(* Logix 5000 AddOnInstructionDefinition export AMCI_SMD34E2_Axis_Follower_Linear; software revision 20.03 *)

ADD_ON_INSTRUCTION AMCI_SMD34E2_Axis_Follower_Linear   (* revision 5.0, vendor AMCI, ExecuteEnableInFalse *)
// Revision note:
// Version 5.0  unlatches the error bit if the rung goes false.  Also modified the Axis Follower commands to by default use the jog CCW command and have an option of the jog CW command.  (The status bits of the jog CCW update faster and the jog CW has smoother motion.)
// Help:
// 2/2017: V0 is the initial release
// 7/2017: V1 added enable and error bits.
// 5/2019: V2 added unlatching the error bit when the rung goes false and the ability to select between normal (jog CCW) and continuous follower (jog CW)
VAR_OUTPUT
   EN : BOOL; {visible}
END_VAR
VAR_INPUT
   Axis_Status_Bits : INT; {required}
   _0_for_Normal_1_for_Continuous : BOOL;
   _0_follow_motor_1_follow_encoder : BOOL;
   Follower_Position : REAL; {required}
   Follower_Velocity : REAL; {required}
   Acceleration : INT; {required}
   Deceleration : INT; {required}
   Proportional_Coefficient : INT; {required}
   Network_delay : INT; {required}
END_VAR
VAR_OUTPUT
   Axis_Follower_occurring : BOOL; {visible}
END_VAR
VAR_IN_OUT
   AMCI_SMD34E2_output_data : _000A:SMD34E2_788832CB:O:0; {required}
END_VAR
VAR_OUTPUT
   ER : BOOL; {visible}
END_VAR
VAR
   command_data_block : INT[10];
        [0]   // Command Bits MSW
        [1]   // Command Bits LSW
        [2]   // Upper Target Position
        [3]   // Lower Target Position
        [4]   // Upper Programmed Speed
        [5]   // Lower Programmed Speed
   axis_follower_position : DINT;
   axis_follower_velocity : DINT;
END_VAR

ROUTINE EnableInFalse   (* ladder *)
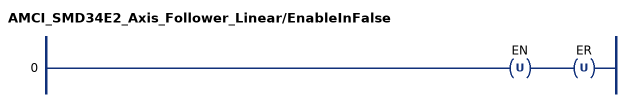
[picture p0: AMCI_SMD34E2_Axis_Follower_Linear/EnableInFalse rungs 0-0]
   0: OTU(EN)OTU(ER);
END_ROUTINE

ROUTINE Logic   (* ladder *)
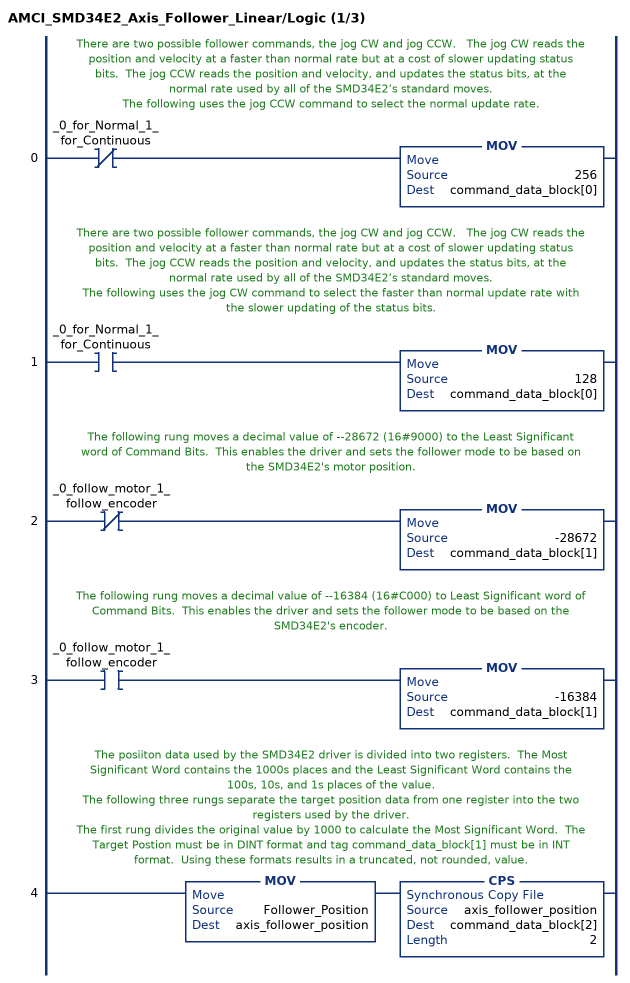
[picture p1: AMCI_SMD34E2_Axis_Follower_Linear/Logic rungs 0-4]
   // There are two possible follower commands, the jog CW and jog CCW.   The jog CW reads the position and velocity at a faster than normal rate but at a cost of slower updating status bits.  The jog CCW reads the position and velocity, and updates the status bits, at the normal rate used by all of the SMD34E2’s standard moves.
   // The following uses the jog CCW command to select the normal update rate.
   0: XIO(_0_for_Normal_1_for_Continuous)MOV(256,command_data_block[0]);
   // There are two possible follower commands, the jog CW and jog CCW.   The jog CW reads the position and velocity at a faster than normal rate but at a cost of slower updating status bits.  The jog CCW reads the position and velocity, and updates the status bits, at the normal rate used by all of the SMD34E2’s standard moves.
   // The following uses the jog CW command to select the faster than normal update rate with the slower updating of the status bits.
   1: XIC(_0_for_Normal_1_for_Continuous)MOV(128,command_data_block[0]);
   // The following rung moves a decimal value of --28672 (16#9000) to the Least Significant word of Command Bits.  This enables the driver and sets the follower mode to be based on the SMD34E2's motor position.
   2: XIO(_0_follow_motor_1_follow_encoder)MOV(-28672,command_data_block[1]);
   // The following rung moves a decimal value of --16384 (16#C000) to Least Significant word of Command Bits.  This enables the driver and sets the follower mode to be based on the SMD34E2's encoder.
   3: XIC(_0_follow_motor_1_follow_encoder)MOV(-16384,command_data_block[1]);
   // The posiiton data used by the SMD34E2 driver is divided into two registers.  The Most Significant Word contains the 1000s places and the Least Significant Word contains the 100s, 10s, and 1s places of the value.
   // The following three rungs separate the target position data from one register into the two registers used by the driver.
   // The first rung divides the original value by 1000 to calculate the Most Significant Word.  The Target Postion must be in DINT format and tag command_data_block[1] must be in INT format.  Using these formats results in a truncated, not rounded, value.
   4: MOV(Follower_Position,axis_follower_position)CPS(axis_follower_position,command_data_block[2],2);
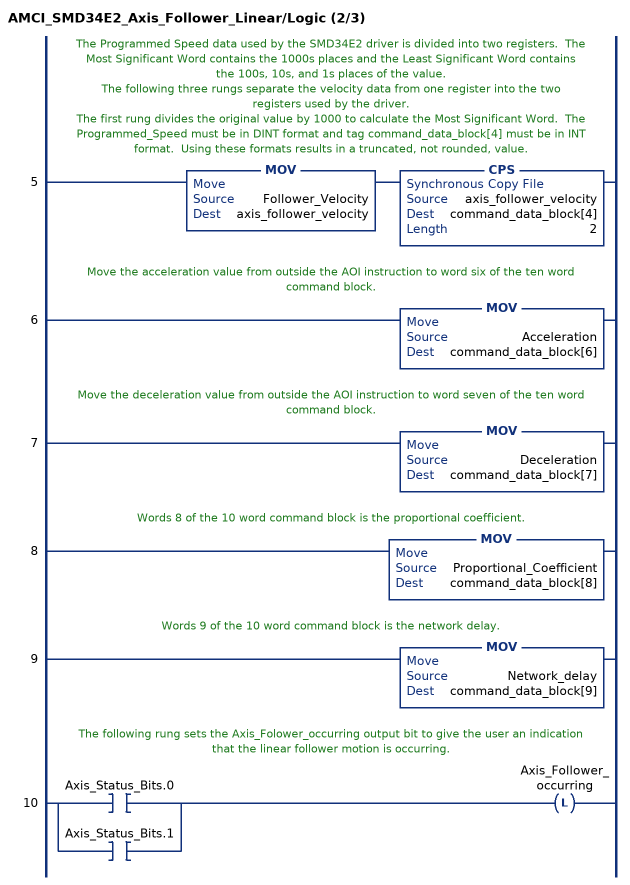
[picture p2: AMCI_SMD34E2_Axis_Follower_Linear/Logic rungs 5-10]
   // The Programmed Speed data used by the SMD34E2 driver is divided into two registers.  The Most Significant Word contains the 1000s places and the Least Significant Word contains the 100s, 10s, and 1s places of the value.
   // The following three rungs separate the velocity data from one register into the two registers used by the driver.
   // The first rung divides the original value by 1000 to calculate the Most Significant Word.  The Programmed_Speed must be in DINT format and tag command_data_block[4] must be in INT format.  Using these formats results in a truncated, not rounded, value.
   5: MOV(Follower_Velocity,axis_follower_velocity)CPS(axis_follower_velocity,command_data_block[4],2);
   // Move the acceleration value from outside the AOI instruction to word six of the ten word command block.
   6: MOV(Acceleration,command_data_block[6]);
   // Move the deceleration value from outside the AOI instruction to word seven of the ten word command block.
   7: MOV(Deceleration,command_data_block[7]);
   // Words 8 of the 10 word command block is the proportional coefficient.
   8: MOV(Proportional_Coefficient,command_data_block[8]);
   // Words 9 of the 10 word command block is the network delay.
   9: MOV(Network_delay,command_data_block[9]);
   // The following rung sets the Axis_Folower_occurring output bit to give the user an indication that the linear follower motion is occurring.
   10: [XIC(Axis_Status_Bits.0) ,XIC(Axis_Status_Bits.1) ]OTL(Axis_Follower_occurring);
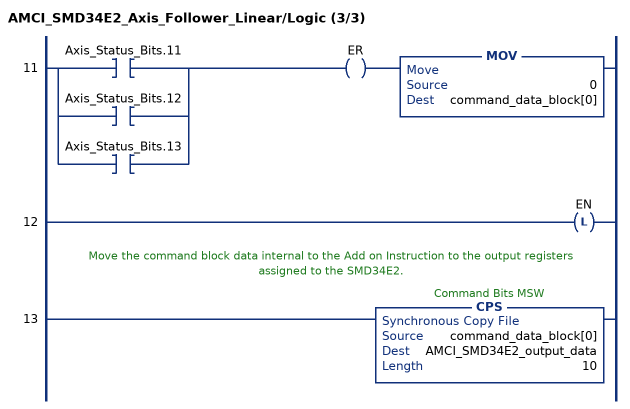
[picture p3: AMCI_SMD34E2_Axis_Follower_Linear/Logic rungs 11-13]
   11: [XIC(Axis_Status_Bits.11) ,XIC(Axis_Status_Bits.12) ,XIC(Axis_Status_Bits.13) ]OTE(ER)MOV(0,command_data_block[0]);
   12: OTL(EN);
   // Move the command block data internal to the Add on Instruction to the output registers assigned to the SMD34E2.
   13: CPS(command_data_block[0],AMCI_SMD34E2_output_data,10);
END_ROUTINE
END_ADD_ON_INSTRUCTION
